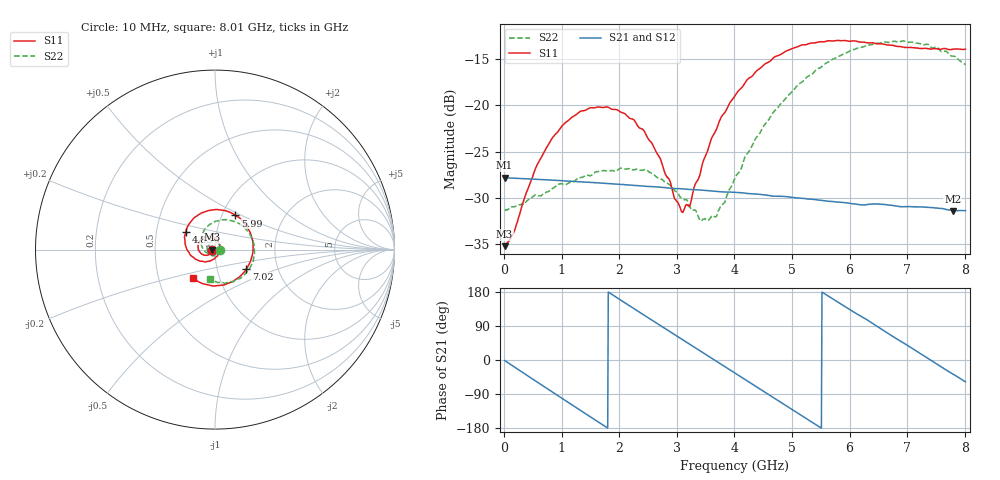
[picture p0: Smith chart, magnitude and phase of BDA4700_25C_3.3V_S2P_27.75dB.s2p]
!Agilent Technologies,E5071B,MY42404982,A.09.10
!Date: Mon Oct 20 18:14:44 2025
!Data & Calibration Information:
!Freq	S11:SOLT2(ON)	S21:SOLT2(ON)	S12:SOLT2(ON)	S22:SOLT2(ON)
# Hz S RI R 50
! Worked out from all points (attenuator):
!   801 points, 10 MHz to 8.01 GHz, reference 50 ohm
!   highest |S21| = -27.81 dB at 10 MHz (marker M1); lowest = -31.4 dB at 7.79 GHz (marker M2)
!   lowest |S11| = -35.2 dB at 10 MHz (marker M3), VSWR 1.04, Z = 48.3 - j0.0922 ohm
!   |S11| at or under -10 dB: start of sweep to end of sweep
!   |S22| runs from -32.5 to -13.0 dB; largest |S21 - S12| = 0.0005
!   S11 on the Smith chart (normalised r, x): 10 MHz: 0.97, -0.00; 4.83 GHz: 0.71, +0.15; 5.99 GHz: 1.16, +0.46; 7.02 GHz: 1.38, -0.31; 8.01 GHz: 0.75, -0.25
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1e7  -0.0173 -0.000954  0.0407 -0.000888  0.0407 -0.0009  0.0271 -0.000811
1.6e8  -0.0179 -0.00946  0.0387 -0.0115  0.0387 -0.0114  0.0272 -0.00769
5.4e8  -0.0347 -0.0288  0.0231 -0.0325  0.023 -0.0325  0.0163 -0.0283
7.4e8  -0.0498 -0.0322  0.0105 -0.0382  0.0106 -0.0381  0.00359 -0.0338
1.35e9  -0.0933 0.00252  -0.0274 -0.0271  -0.0274 -0.0272  -0.0364 -0.0183
2.09e9  -0.0544 0.0722  -0.0329 0.0176  -0.0329 0.0176  -0.0297 0.0342
2.42e9  -0.0129 0.0724  -0.018 0.0319  -0.018 0.0319  -0.00527 0.0444
2.68e9  0.0146 0.0515  -0.00258 0.0361  -0.00261 0.0361  0.0127 0.0383
3.11e9  0.0259 -0.00604  0.0216 0.0279  0.0214 0.0281  0.0288 0.0111
3.23e9  0.0199 -0.021  0.0265 0.023  0.0265 0.023  0.0279 0.00291
3.55e9  -0.0149 -0.0569  0.0341 0.00596  0.0341 0.00589  0.0131 -0.02
3.7e9  -0.0396 -0.0648  0.0341 -0.00271  0.0341 -0.00281  0.000356 -0.0257
4.01e9  -0.0961 -0.0589  0.0279 -0.0192  0.0279 -0.0191  -0.0309 -0.0259
4.37e9  -0.1516 -0.00767  0.0117 -0.0311  0.0117 -0.0311  -0.0664 0.00199
4.83e9  -0.1627 0.1  -0.0131 -0.0294  -0.0129 -0.0294  -0.0764 0.0707
5.35e9  -0.0728 0.2047  -0.0299 -0.00828  -0.0299 -0.00846  -0.0159 0.1467
5.99e9  0.1142 0.1906  -0.0206 0.0212  -0.0208 0.0211  0.1282 0.1476
6.68e9  0.2118 -0.000719  0.0104 0.0269  0.0105 0.027  0.2192 0.000791
7.02e9  0.1752 -0.1083  0.0226 0.0171  0.0227 0.017  0.2 -0.0903
7.45e9  0.0583 -0.1941  0.0279 -0.00213  0.0279 -0.00217  0.1131 -0.1701
7.79e9  -0.0571 -0.1928  0.0215 -0.0161  0.0216 -0.0163  0.0227 -0.183
8.01e9  -0.1222 -0.1602  0.0145 -0.0228  0.0146 -0.0227  -0.0299 -0.163
